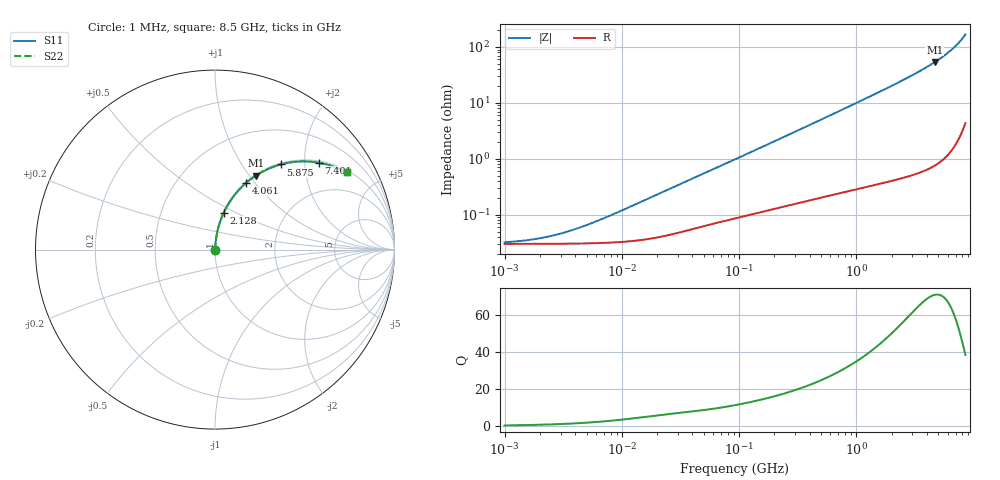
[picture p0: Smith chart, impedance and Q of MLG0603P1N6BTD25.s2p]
! S-Parameter Data Generated by TDK Corporation
! Copyright(C) 2025 TDK Corporation.
! All Rights Reserved.
! TDK P/N: MLG0603P1N6BTD25 (SMD / SMT Inductor (Coil))
! Property: L=1.6nH at 500MHz
! Size(LxWxT): 0.6x0.3x0.3mm
! Model Type: s2p (Touchstone File Format Version 1.0)
! Frequency: DC=Yes Start=1MHz Stop=8500MHz 198points Log-sweep
! Model Generated on Feb. 6, 2025
! Terms and conditions regarding TDK Simulation Models:
! 1)This simulation model is being provided solely for informational
!  purposes. Please refer to the specifications of the products in
!  terms of detailed characteristics of such products.
! 2)In no event shall TDK Corporation of any of its subsidiaries be
!  liable for any loss or damage arising, directly or indirectly,
!  from any information contained in this simulation model, including,
!  but not limited to loss or damages arising from any inaccuracies,
!  omissions or errors in connection with such information.
! 3)Any and all copyrights on this simulation model are owned by
!  TDK Corporation.  Duplication or redistribution of this simulation
!  model without prior written permission from TDK Corporation
!  is prohibited.
! 4)This simulation model is subject to any modification or change
!  without any prior notice.
! 5)Neither TDK Corporation nor any of its subsidiaries shall make any
!  warranty, express or implied, including but not limited to the
!  correctness, implied warranties of merchantability and fitness for
!  a particular purpose with respect to this simulation models.
! 6)The use of this simulation model shall be deemed to have consented
!  to the terms and conditions hereof.
! Port Assignments:
!  1 ---@@@--- 2
! Applicable Conditions:
!  Temperature = 25 degC
!  DC Bias Current = 0 A
!  Small Signal Operation
# Hz S MA R 50
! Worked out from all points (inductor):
!   197 points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, 1 MHz to 8.5 GHz, reference 50 ohm
!   read as one part in series: L = 1.83 nH near 8.36 MHz
!   highest Q = 71.1 at 4.664 GHz (marker M1), where L = 1.84 nH
!   S11 on the Smith chart (normalised r, x): 1 MHz: 1.00, +0.00; 2.128 GHz: 1.01, +0.43; 4.061 GHz: 1.01, +0.90; 5.875 GHz: 1.02, +1.51; 7.401 GHz: 1.04, +2.34; 8.5 GHz: 1.09, +3.36
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1000000  0.0003215 21.0  0.9997 -0.0  0.9997 -0.0  0.0003215 21.0
1515069  0.0003476 30.1  0.9997 -0.0  0.9997 -0.0  0.0003476 30.1
2191881  0.0003931 40.0  0.9997 -0.0  0.9997 -0.0  0.0003931 40.0
3171038  0.0004743 50.3  0.9997 -0.0  0.9997 -0.0  0.0004743 50.3
4587603  0.0006102 59.9  0.9997 -0.0  0.9997 -0.0  0.0006102 59.9
8360083  0.001012 71.6  0.9997 -0.1  0.9997 -0.1  0.001012 71.6
2.10461e7  0.002414 80.3  0.9996 -0.1  0.9996 -0.1  0.002414 80.3
9.219544e7  0.009771 84.4  0.9991 -0.6  0.9991 -0.6  0.009771 84.4
4.229561e8  0.04257 85.1  0.9972 -2.4  0.9972 -2.4  0.04257 85.1
9.708683e8  0.09627 82.8  0.9926 -5.5  0.9926 -5.5  0.09627 82.8
1.404574e9  0.1388 80.7  0.987 -8.0  0.987 -8.0  0.1388 80.7
1.940355e9  0.1917 77.8  0.9776 -11.0  0.9776 -11.0  0.1917 77.8
2.128028e9  0.2103 76.8  0.9736 -12.1  0.9736 -12.1  0.2103 76.8
3.07866e9  0.3061 71.3  0.9471 -17.8  0.9471 -17.8  0.3061 71.3
4.061159e9  0.4076 65.1  0.9073 -24.1  0.9073 -24.1  0.4076 65.1
4.664383e9  0.471 61.1  0.8755 -28.1  0.8755 -28.1  0.471 61.1
5.357206e9  0.5445 56.2  0.8311 -33.0  0.8311 -33.0  0.5445 56.2
5.87536e9  0.5993 52.3  0.7918 -36.8  0.7918 -36.8  0.5993 52.3
6.748056e9  0.6896 45.5  0.7129 -43.6  0.7129 -43.6  0.6896 45.5
7.400733e9  0.7537 40.0  0.6432 -48.9  0.6432 -48.9  0.7537 40.0
8.116539e9  0.8182 33.8  0.5565 -54.9  0.5565 -54.9  0.8182 33.8
8.5e9  0.8495 30.4  0.5061 -58.1  0.5061 -58.1  0.8495 30.4
